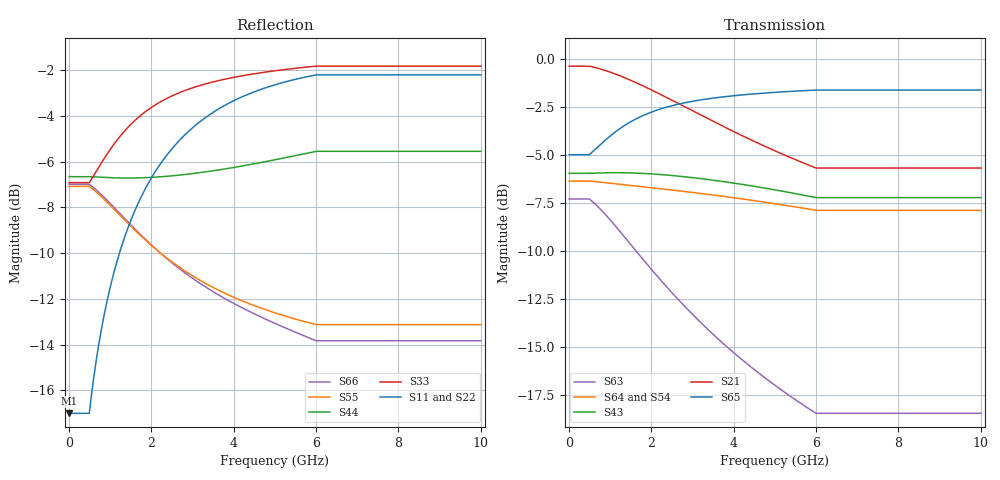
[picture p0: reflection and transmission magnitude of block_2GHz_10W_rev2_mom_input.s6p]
! Created Wed May 20 10:28:38 2015
# ghz S ma R 50
! 6 Port Network Data from SP1.SP block
! freq  magS11  angS11  magS12  angS12  magS13  angS13  magS14  angS14
!  magS15  angS15  magS16  angS16
!  magS21  angS21  magS22  angS22
!  magS23  angS23  magS24  angS24  magS25  angS25  magS26  angS26
!  magS31  angS31  magS32  angS32  magS33  angS33  magS34  angS34
!  magS35  angS35  magS36  angS36
!  magS41  angS41  magS42  angS42
!  magS43  angS43  magS44  angS44  magS45  angS45  magS46  angS46
!  magS51  angS51  magS52  angS52  magS53  angS53  magS54  angS54
!  magS55  angS55  magS56  angS56
!  magS61  angS61  magS62  angS62
!  magS63  angS63  magS64  angS64  magS65  angS65  magS66  angS66
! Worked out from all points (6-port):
!   1000 points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, 10 MHz to 10 GHz, reference 50 ohm
!   strongest paths, dB at 10 MHz, 2.51 GHz, 5.01 GHz, 7.51 GHz, 10 GHz:
!     S65: -5.0, -2.4, -1.7, -1.6, -1.6
!     S21: -0.4, -2.2, -4.8, -5.7, -5.7
!     S43: -6.0, -6.1, -6.8, -7.2, -7.2
!     S64: -6.4, -6.8, -7.5, -7.9, -7.9
!     S54: -6.4, -6.9, -7.8, -8.2, -8.2
!     S63: -7.3, -12.2, -17.0, -18.5, -18.5
!   lowest |S11| = -17.0 dB at 10 MHz (marker M1), VSWR 1.33, Z = 53.9 + j14.3 ohm
!   |S11| at or under -10 dB: start of sweep to 1.231 GHz
